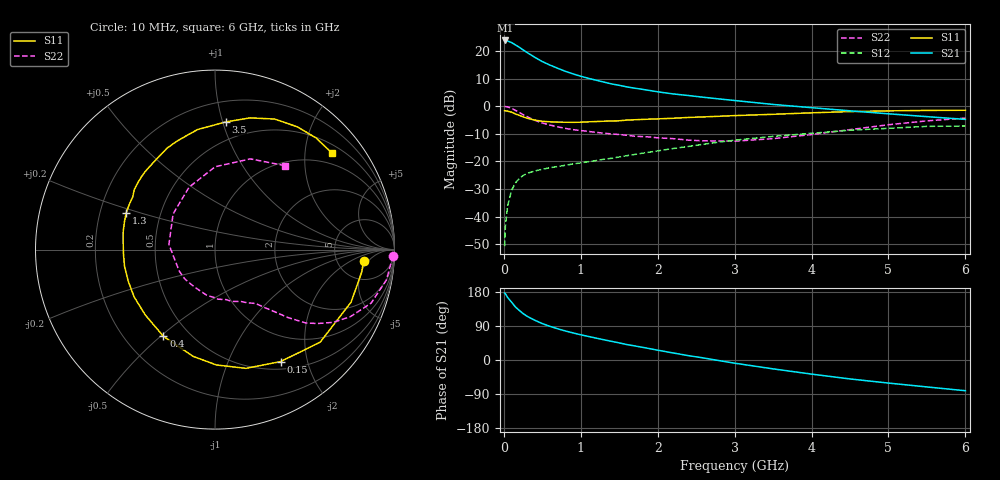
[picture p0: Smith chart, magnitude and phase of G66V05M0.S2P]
! SIEMENS Small Signal Semiconductors
! BFG193
! Si NPN RF Bipolar Junction Transistor in SOT223
! VCE = 6 V  IC = 5 mA
! Common Emitter S-Parameters:  August  1996
# GHz  S  MA  R  50
!  f  S11  S21  S12  S22
! GHz  MAG  ANG  MAG  ANG  MAG  ANG  MAG  ANG
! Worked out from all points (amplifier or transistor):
!   36 points, 10 MHz to 6 GHz, reference 50 ohm
!   highest |S21| = 23.9 dB at 20 MHz (marker M1)
!   |S21| within 3 dB of that: start of sweep to 228.7 MHz
!   unconditionally stable (mu >= 1): 1.131 GHz to 2.494 GHz
!   at 250 MHz: K = 0.33, MSG = 22.8 dB, |S12| = -25.1 dB
!   at 1.4 GHz: K = 1.08, MAG = 11.8 dB, |S12| = -18.9 dB
!   at 6 GHz: K = 0.87, MSG = 1.2 dB, |S12| = -7.2 dB
!   S11 on the Smith chart (normalised r, x): 10 MHz: 9.27, -3.71; 150 MHz: 0.60, -1.58; 400 MHz: 0.36, -0.51; 1.3 GHz: 0.31, +0.18; 3.5 GHz: 0.35, +1.02; 6 GHz: 0.70, +2.63
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0.01  0.8301 -4.3  15.51 176.8  0.0029 89.8  0.9921 -2.0
0.02  0.8271 -8.7  15.58 174.7  0.0067 85.9  0.985 -4.0
0.05  0.8127 -21.1  15.23 164.7  0.0158 79.0  0.9701 -10.0
0.1  0.7806 -41.3  14.27 152.8  0.0297 69.9  0.9196 -18.9
0.15  0.7232 -59.6  12.96 140.0  0.0406 61.2  0.8423 -26.3
0.2  0.6837 -75.4  11.74 131.1  0.0489 55.3  0.7737 -31.6
0.25  0.6428 -89.3  10.52 122.5  0.0553 50.3  0.7024 -35.9
0.3  0.6069 -101.7  9.462 115.6  0.0605 46.9  0.649 -39.0
0.4  0.562 -120.8  7.744 105.2  0.0669 42.6  0.5567 -42.9
0.5  0.5324 -136.9  6.445 96.0  0.0719 39.9  0.4963 -45.4
0.6  0.522 -149.7  5.57 88.8  0.0767 39.0  0.4551 -47.5
0.7  0.5144 -160.2  4.875 82.4  0.0806 39.0  0.423 -49.6
0.9  0.5106 -177.4  3.855 71.4  0.0898 38.8  0.3765 -53.0
1.1  0.5211 169.0  3.201 62.1  0.0987 39.6  0.3486 -58.3
1.3  0.5351 157.8  2.741 53.4  0.1094 39.8  0.3238 -63.3
1.6  0.561 143.2  2.239 40.7  0.1269 39.2  0.2972 -73.9
2.2  0.6048 121.2  1.671 18.6  0.171 34.6  0.2585 -100.2
2.8  0.6577 103.0  1.355 -1.7  0.2238 25.8  0.2345 -135.9
3.5  0.7137 85.2  1.077 -23.4  0.2839 11.2  0.2583 173.8
4.5  0.7995 65.5  0.825 -50.0  0.3675 -9.5  0.3765 112.6
5.5  0.839 47.8  0.647 -71.1  0.4311 -35.7  0.5424 68.7
6  0.8452 39.4  0.577 -81.1  0.4384 -50.6  0.6095 50.1
